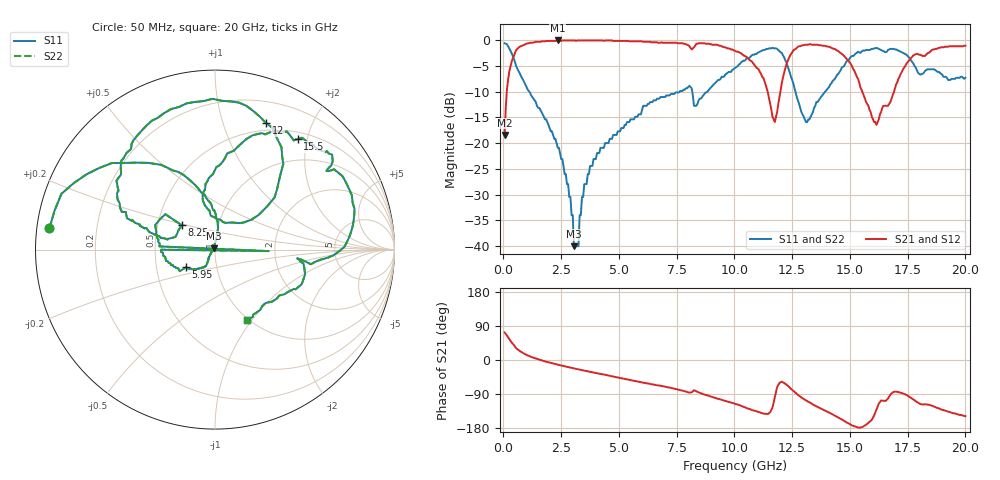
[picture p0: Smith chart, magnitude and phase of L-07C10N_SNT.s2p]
#	mhz	s	ma	r	50
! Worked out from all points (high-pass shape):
!   400 points, 50 MHz to 20 GHz, reference 50 ohm
!   highest |S21| = -0.09 dB at 2.35 GHz (marker M1); lowest = -18.4 dB at 50 MHz (marker M2)
!   |S21| within 3 dB of the highest: 450.9 MHz to 10.45 GHz (9.995 GHz wide, 183 % of centre); 12.4 GHz to 14.75 GHz (2.346 GHz wide, 17.3 % of centre)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
!   lowest |S11| = -40.0 dB at 3.05 GHz (marker M3), VSWR 1.02, Z = 49.4 + j0.777 ohm
!   |S11| at or under -10 dB: 1.119 GHz to 7.631 GHz (6.513 GHz wide, 149 % of centre); 8.173 GHz to 8.831 GHz (658.5 MHz wide, 7.75 % of centre); 12.64 GHz to 13.93 GHz (1.292 GHz wide, 9.73 % of centre)
!   |S22| runs from -40.0 to -0.6 dB; largest |S21 - S12| = 0
!   S11 on the Smith chart (normalised r, x): 50 MHz: 0.04, +0.06; 5.95 GHz: 0.71, -0.15; 8.25 GHz: 0.67, +0.19; 12 GHz: 0.42, +1.40; 15.5 GHz: 0.61, +1.84; 20 GHz: 0.99, -0.95
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50  0.93 172.7  0.12 72.7  0.12 72.7  0.93 172.7
550  0.56 122.5  0.8 31.1  0.8 31.1  0.56 122.5
2350  0.09 81.5  0.99 -12.2  0.99 -12.2  0.09 81.5
3050  0.01 128.1  0.99 -22.0  0.99 -22.0  0.01 128.1
3400  0.03 -140.0  0.99 -26.8  0.99 -26.8  0.03 -140.0
5950  0.19 -148.6  0.97 -58.3  0.97 -58.3  0.19 -148.6
6700  0.27 -165.2  0.94 -67.0  0.94 -67.0  0.27 -165.2
7350  0.3 -179.9  0.94 -74.9  0.94 -74.9  0.3 -179.9
7400  0.3 -1.6  0.94 -75.6  0.94 -75.6  0.3 -1.6
7450  0.31 176.7  0.94 -76.2  0.94 -76.2  0.31 176.7
8250  0.23 143.8  0.85 -79.8  0.85 -79.8  0.23 143.8
10050  0.54 157.1  0.78 -116.3  0.78 -116.3  0.54 157.1
11050  0.76 126.7  0.52 -137.6  0.52 -137.6  0.76 126.7
11750  0.83 84.0  0.16 -98.2  0.16 -98.2  0.83 84.0
12000  0.76 68.0  0.33 -58.8  0.33 -58.8  0.76 68.0
12600  0.34 39.1  0.81 -84.4  0.81 -84.4  0.34 39.1
13350  0.19 97.2  0.9 -115.7  0.9 -115.7  0.19 97.2
14500  0.47 87.0  0.78 -152.1  0.78 -152.1  0.47 87.0
15500  0.77 53.2  0.33 -177.6  0.33 -177.6  0.77 53.2
16700  0.81 31.9  0.24 -96.5  0.24 -96.5  0.81 31.9
17750  0.59 -5.5  0.71 -103.9  0.71 -103.9  0.59 -5.5
20000  0.43 -65.4  0.88 -148.3  0.88 -148.3  0.43 -65.4
